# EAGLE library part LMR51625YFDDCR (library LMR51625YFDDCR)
Functional Safety-Capable Documentation available to aid functional safety system design Configured for rugged industrial applications: 4.3V to 60V input voltage range 2.5A or 3.5A continuous output current Low operating quiescent current of 29uA 70ns minimum switching on time 400kHz amd 1.1MHz switching frequency Frequency spread spectrum (PFM variant) 40C to 150C junction temperature range 96% maximum duty cycle Monotonic start-up with prebiased output Short-circu Source: Datasheet
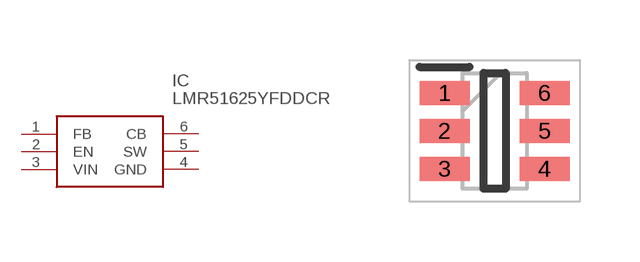
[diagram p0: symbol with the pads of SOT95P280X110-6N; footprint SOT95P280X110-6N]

Designator prefix IC

## LMR51625YFDDCR (Arrow_Part_Number: LMR51625YFDDCR; Arrow_Price-Stock: https://www.arrow.com/en/products/lmr51625yfddcr/texas-instruments?utm_currency=USD&region=nac; Description: Functional Safety-Capable Documentation available to aid functional safety system design Configured for rugged industrial applications: 4.3V to 60V input voltage range 2.5A or 3.5A continuous output current Low operating quiescent current of 29uA 70ns minimum switching on time 400kHz amd 1.1MHz switching frequency Frequency spread spectrum (PFM variant) 40C to 150C junction temperature range 96% maximum duty cycle Monotonic start-up with prebiased output Short-circu; Height: 1.1mm; Manufacturer_Name: Texas Instruments; Manufacturer_Part_Number: LMR51625YFDDCR; Mouser_Part_Number: 595-LMR51625YFDDCR; Mouser_Price-Stock: https://www.mouser.co.uk/ProductDetail/Texas-Instruments/LMR51625YFDDCR?qs=efUn273yAhe0Di9PgWnVVg%3D%3D)  [SOT95P280X110-6N]
1  FB
2  EN
3  VIN
4  GND
5  SW
6  CB

## Footprint SOT95P280X110-6N (pad centres in mm)
DDC0006A
smd 1.25 x 0.6: 1 -1.25,0.95; 2 -1.25,0; 3 -1.25,-0.95; 4 1.25,-0.95; 5 1.25,0; 6 1.25,0.95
